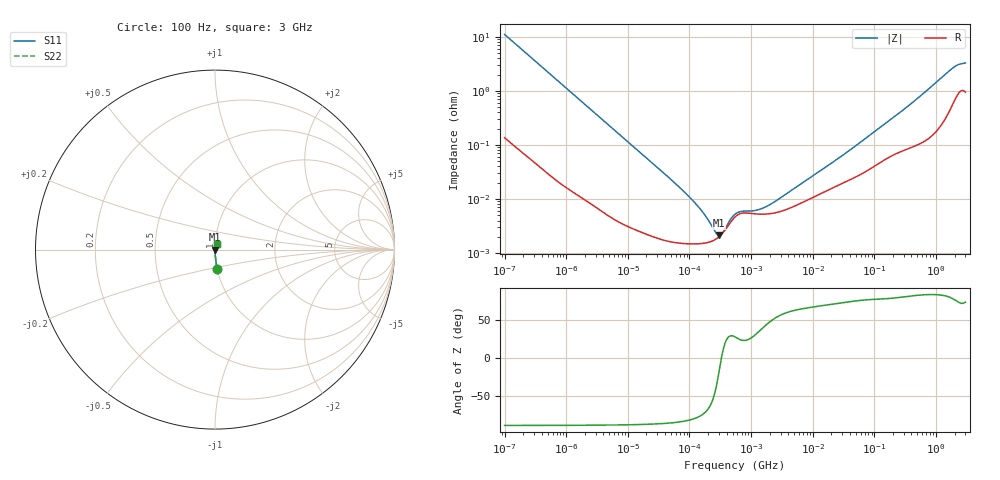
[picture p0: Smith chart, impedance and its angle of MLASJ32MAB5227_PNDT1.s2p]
! MLASJ32MAB5227_PNDT1  S-PARAMETER MODEL  ( Standard Model )
! Model Generated by TAIYO YUDEN Corporation (https://www.yuden.co.jp/en/)
! Version 2.0
! TAIYO YUDEN Control No. 250312
! Copyright(c) 2013 TAIYO YUDEN CO.,LTD. All Rights Reserved.
! Product Description (link to TY-COMPAS)
! https://ds.yuden.co.jp/TYCOMPAS/or/detail?pn=MLASJ32MAB5227MPNDT1&u=M
! Products Name : Multilayer Ceramic Capacitors
! Characteristics :
!  Capacitance : 220 [uF] , Rated Voltage : 6.3 [V] , TCC : X5R
!  Case Size : 3.2 x 2.5 / 0.126 x 0.098 [mm/inch] , Thickness : 2.5 / 0.098 [mm/inch]
!  (Conditions: Temperature = 25 [degC] , DC Bias Voltage = 0 [V])
! External Node Assignments :
!  1  o---| |---o  2
! GND o---------o GND
! Frequency Range : 100Hz  -  3GHz  [ 401 STEP ]
# MHZ S RI R 50
! Freq[MHz].  S11 Real  S11 Imag  S21 Real  S21 Imag  S12 Real  S12 Imag  S22 Real  S22 Imag
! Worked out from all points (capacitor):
!   401 points, 100 Hz to 3 GHz, reference 50 ohm
!   read as one part in series: C = 144 uF near 109 Hz
!   lowest |Z| = 2.11 mohm at 299.8 kHz (marker M1)
!   series resonance near 330.9 kHz, so ESL is about 1.6 nH
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0.0001  0.0134 -0.1088  0.9866 0.1088  0.9866 0.1088  0.0134 -0.1088
0.000114  0.0105 -0.096  0.9895 0.096  0.9895 0.096  0.0105 -0.096
0.000175  0.00479 -0.063  0.9952 0.063  0.9952 0.063  0.00479 -0.063
0.000306  0.00179 -0.0363  0.9982 0.0363  0.9982 0.0363  0.00179 -0.0363
0.001788  0.000145 -0.00632  0.9999 0.00632  0.9999 0.00632  0.000145 -0.00632
0.031977  1.85e-05 -0.000361  1 0.000361  1 0.000361  1.85e-05 -0.000361
0.060986  1.55e-05 -0.000186  1 0.000186  1 0.000186  1.55e-05 -0.000186
0.097915  1.48e-05 -0.00011  1 0.00011  1 0.00011  1.48e-05 -0.00011
0.106717  1.48e-05 -9.94e-05  1 9.94e-05  1 9.94e-05  1.48e-05 -9.94e-05
0.116311  1.48e-05 -8.94e-05  1 8.94e-05  1 8.94e-05  1.48e-05 -8.94e-05
0.299821  1.99e-05 -7.19e-06  1 7.19e-06  1 7.19e-06  1.99e-05 -7.19e-06
0.547723  4.64e-05 2.4e-05  1 -2.4e-05  1 -2.4e-05  4.64e-05 2.4e-05
2.579298  5.62e-05 7.49e-05  0.9999 -7.49e-05  0.9999 -7.49e-05  5.62e-05 7.49e-05
2.81117  5.76e-05 8.17e-05  0.9999 -8.17e-05  0.9999 -8.17e-05  5.76e-05 8.17e-05
3.063887  5.92e-05 8.89e-05  0.9999 -8.89e-05  0.9999 -8.89e-05  5.92e-05 8.89e-05
9.794414  0.000105 0.000242  0.9999 -0.000242  0.9999 -0.000242  0.000105 0.000242
35.62563  0.000213 0.000696  0.9998 -0.000696  0.9998 -0.000696  0.000213 0.000696
175.1444  0.000602 0.00278  0.9994 -0.00278  0.9994 -0.00278  0.000602 0.00278
451.4794  0.000991 0.0065  0.999 -0.0065  0.999 -0.0065  0.000991 0.0065
1868.531  0.00625 0.0255  0.9937 -0.0255  0.9937 -0.0255  0.00625 0.0255
2317.205  0.00971 0.0288  0.9903 -0.0288  0.9903 -0.0288  0.00971 0.0288
3000  0.0103 0.0308  0.9897 -0.0308  0.9897 -0.0308  0.0103 0.0308
